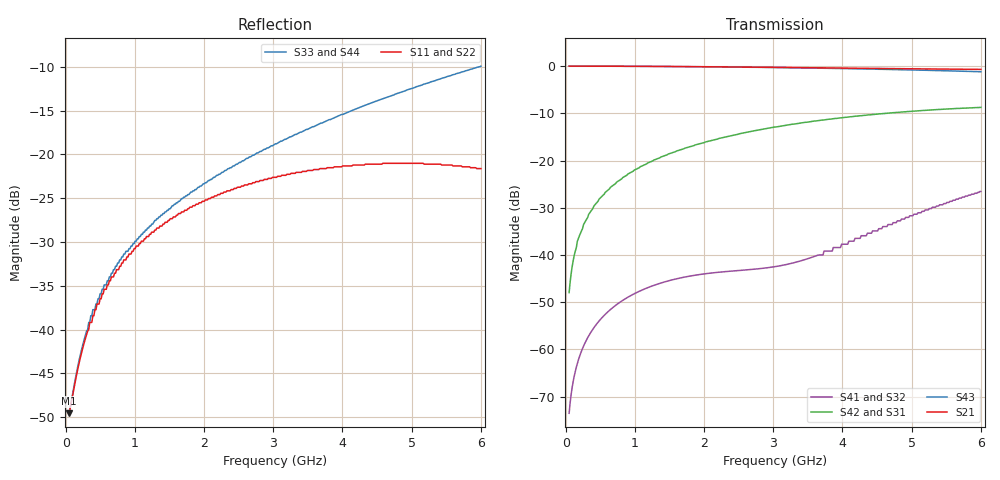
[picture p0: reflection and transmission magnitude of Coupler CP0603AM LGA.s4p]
!	AVX THIN FILM OPERATION
!	CP0603 HIGH DIRECTIVITY COUPLERS
!	P/N CP0603AxxxxMLTR
!	Network	Analyzer HP8720ES.07.64:Feb23,2000 Serial No.US39172382
!	Hewlett-Packard
!	24 July 2003	02:45:57
# MHZ S MA R 50
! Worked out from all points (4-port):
!   400 points, 50 MHz to 6 GHz, reference 50 ohm
!   strongest paths, dB at 50 MHz, 1.541 GHz, 3.032 GHz, 4.524 GHz, 6 GHz:
!     S21: 0.0, -0.1, -0.3, -0.5, -0.7
!     S43: 0.0, -0.1, -0.3, -0.7, -1.2
!     S42: -48.0, -18.3, -12.9, -10.1, -8.8
!     S31: -48.0, -18.3, -12.9, -10.1, -8.8
!     S41: -73.5, -45.3, -42.4, -34.4, -26.6
!     S32: -73.5, -45.3, -42.4, -34.4, -26.6
!   lowest |S11| = -49.6 dB at 50 MHz (marker M1), VSWR 1.01, Z = 50.3 - j0.151 ohm
!   |S11| at or under -10 dB: start of sweep to end of sweep
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50  0.00333 -26.7  0.997 -0.5  0.003998 89.4  0.000211 88.9
    0.997 -0.5  0.00333 -26.7  0.000211 88.9  0.003998 89.4
    0.003998 89.4  0.000211 88.9  0.003361 26.7  0.997 -0.6
    0.000211 88.9  0.003998 89.4  0.997 -0.6  0.003361 26.7
169.298  0.005803 -60.8  0.997 -1.6  0.014 88.1  0.000713 87.6
         0.997 -1.6  0.005803 -60.8  0.000713 87.6  0.014 88.1
         0.014 88.1  0.000713 87.6  0.00601 58.3  0.997 -2.1
         0.000713 87.6  0.014 88.1  0.997 -2.1  0.00601 58.3
378.07  0.011 -78.8  0.996 -3.5  0.03 85.9  0.001579 85.4
        0.996 -3.5  0.011 -78.8  0.001579 85.4  0.03 85.9
        0.03 85.9  0.001579 85.4  0.012 71.3  0.996 -4.8
        0.001579 85.4  0.03 85.9  0.996 -4.8  0.012 71.3
661.404  0.02 -87.9  0.995 -6.1  0.053 82.8  0.002702 82.6
         0.995 -6.1  0.02 -87.9  0.002702 82.6  0.053 82.8
         0.053 82.8  0.002702 82.6  0.021 74.0  0.995 -8.3
         0.002702 82.6  0.053 82.8  0.995 -8.3  0.021 74.0
1272.807  0.036 -97.9  0.991 -11.6  0.101 76.2  0.004767 77.7
          0.991 -11.6  0.036 -97.9  0.004767 77.7  0.101 76.2
          0.101 76.2  0.004767 77.7  0.041 70.6  0.991 -16.1
          0.004767 77.7  0.101 76.2  0.991 -16.1  0.041 70.6
3718.421  0.083 -122.2  0.956 -33.1  0.268 50.0  0.01 111.4
          0.956 -33.1  0.083 -122.2  0.01 111.4  0.268 50.0
          0.268 50.0  0.01 111.4  0.152 42.5  0.948 -47.1
          0.01 111.4  0.268 50.0  0.948 -47.1  0.152 42.5
6000  0.083 -141.1  0.922 -51.8  0.365 25.9  0.047 111.0
      0.922 -51.8  0.083 -141.1  0.047 111.0  0.365 25.9
      0.365 25.9  0.047 111.0  0.319 12.9  0.87 -77.0
      0.047 111.0  0.365 25.9  0.87 -77.0  0.319 12.9
